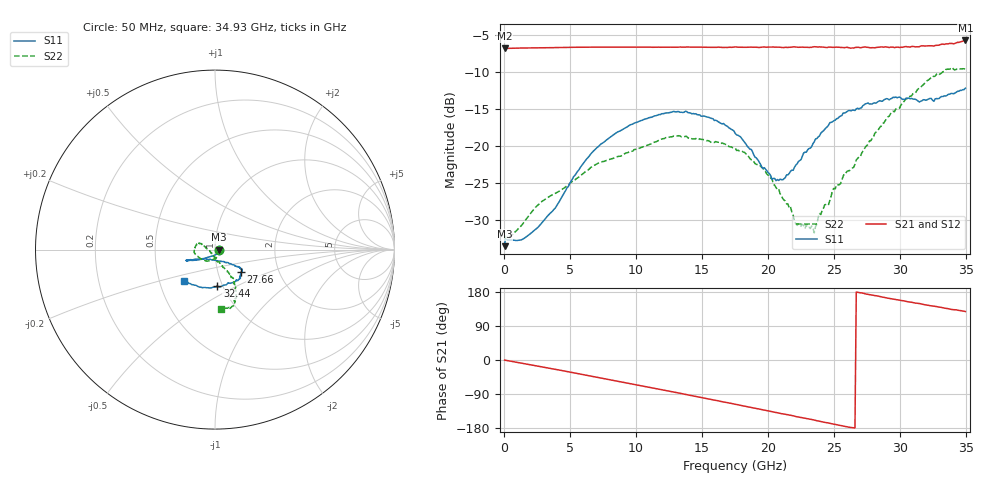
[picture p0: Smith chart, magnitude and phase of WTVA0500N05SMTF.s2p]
! 50 ohm 2-Port S-parameters measured by Modelithics Inc support@modelithics.com  Tampa, FL USA 813-866-6335 (February 2024)
! Smiths Interconnect,  5dB P/N: WTVA0500N05SMTF, Temperature: -25 C
! Board: 10 mil Rogers 4350B, Mounting Pad Dimensions: Length: 15 mils, Width: 25 mils, Gap: 40 mils.
# Hz S RI R 50
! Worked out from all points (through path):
!   352 points, 50 MHz to 34.93 GHz, reference 50 ohm
!   highest |S21| = -5.76 dB at 34.93 GHz (marker M1); lowest = -6.8 dB at 50 MHz (marker M2)
!   group delay of S21, straight-line fit = 18.9 ps
!   lowest |S11| = -33.5 dB at 50 MHz (marker M3), VSWR 1.04, Z = 52.2 - j0.0332 ohm
!   |S11| at or under -10 dB: start of sweep to end of sweep
!   |S22| runs from -32.6 to -9.4 dB; largest |S21 - S12| = 0.0045
!   S11 on the Smith chart (normalised r, x): 50 MHz: 1.04, -0.00; 27.66 GHz: 1.29, -0.34; 32.44 GHz: 0.94, -0.40; 34.93 GHz: 0.67, -0.25
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5e7  0.0211 -0.000318  0.4552 -0.00191  0.4549 -0.0021  0.025 -0.000209
1e8  0.0235 -0.00175  0.4553 -0.00442  0.4549 -0.00443  0.0232 -0.00278
1.2945e9  0.0156 -0.0173  0.4538 -0.0636  0.4534 -0.0636  0.0182 -0.0225
2.588e9  0.00374 -0.0282  0.4411 -0.1287  0.4406 -0.1288  0.0136 -0.0378
5.8715e9  -0.0562 -0.0478  0.3672 -0.2834  0.3668 -0.2835  -0.0232 -0.0597
8.558e9  -0.1089 -0.0591  0.2631 -0.3834  0.2623 -0.3835  -0.0608 -0.0592
1.1742e10  -0.1526 -0.0582  0.1033 -0.4528  0.1023 -0.4528  -0.1056 -0.0306
1.4528e10  -0.1533 -0.0613  -0.0499 -0.4618  -0.0508 -0.4615  -0.1121 0.00968
1.7513e10  -0.1096 -0.0523  -0.2106 -0.4161  -0.2114 -0.4154  -0.0899 0.0355
1.9304e10  -0.0595 -0.0511  -0.2931 -0.3576  -0.294 -0.3566  -0.0705 0.0259
2.05975e10  -0.0155 -0.0563  -0.348 -0.3073  -0.3488 -0.3061  -0.0511 0.0113
2.1692e10  0.0196 -0.0648  -0.3831 -0.261  -0.3835 -0.26  -0.0389 0.00026
2.21895e10  0.0377 -0.066  -0.4012 -0.2333  -0.4017 -0.2321  -0.0285 -0.00642
2.33835e10  0.0734 -0.0733  -0.4308 -0.1776  -0.431 -0.1767  -0.0184 -0.0215
2.3483e10  0.0767 -0.0741  -0.4352 -0.1715  -0.4353 -0.1707  -0.0151 -0.0212
2.3881e10  0.0875 -0.0778  -0.4425 -0.1475  -0.4425 -0.1467  -0.012 -0.0329
2.45775e10  0.1085 -0.0865  -0.4518 -0.1108  -0.4519 -0.1097  -0.0025 -0.0403
2.5672e10  0.1351 -0.0983  -0.459 -0.0461  -0.4588 -0.0453  0.011 -0.0615
2.7662e10  0.1441 -0.1268  -0.4568 0.0621  -0.4564 0.0637  0.0447 -0.0988
2.91545e10  0.1375 -0.1517  -0.4406 0.1377  -0.4399 0.1391  0.081 -0.1368
3.2438e10  0.0135 -0.2033  -0.3751 0.2897  -0.3736 0.2913  0.1145 -0.2734
3.49255e10  -0.1744 -0.173  -0.3171 0.4063  -0.3141 0.4082  0.0362 -0.3288
